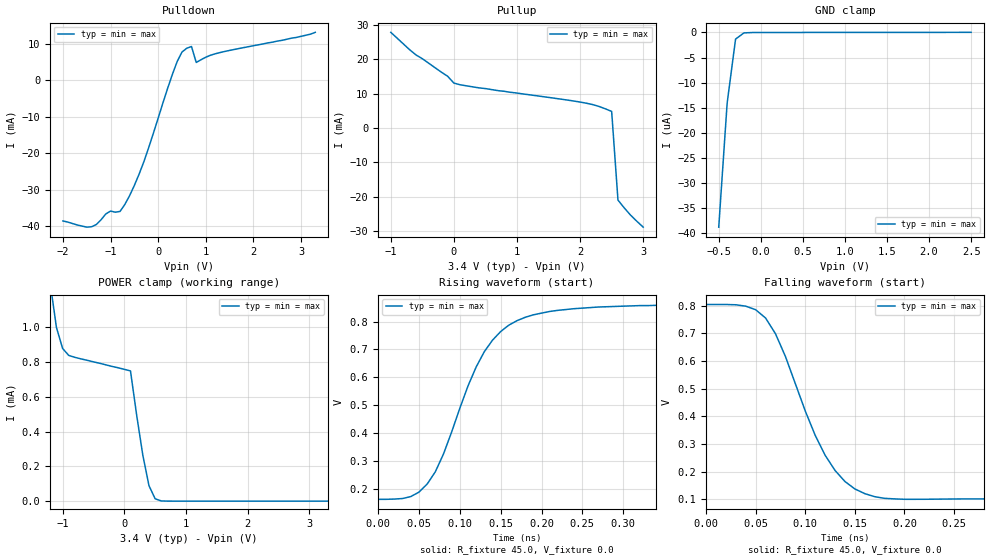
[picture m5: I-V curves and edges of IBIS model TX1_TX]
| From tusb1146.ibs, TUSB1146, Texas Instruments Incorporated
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[Model] TX1_TX
Model_type Output
| typ min max
C_comp 0.949p 0.949p 0.949p
[Algorithmic Model]
Executable Windows_cl19.16.27034_64  TX1_TX_x64.dll TX1_TX.ami
|Executable Windows_cl19.16.27034_64 TX1_x64.dll TX1.ami
|Executable Linux_gcc5.4.0_64 TX1_TX_x64.so TX1_TX.ami
[End Algorithmic Model]
[Temperature_Range] 27 27 27
[Voltage Range] 3.4 3.4 3.4
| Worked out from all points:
|   slope of the pulldown table from 0 to 0.51 V, typ, clamps not added: 28 ohm
|   slope of the pullup table from 0 to 0.51 V, typ, clamps not added: 313 ohm
|   POWER clamp passes 1 mA (typ) near -1.10 V on its own axis
|   rising waveform, R_fixture 45.0, V_fixture 0.0: 20-80 % time 56.8ps typ, 56.8ps min, 56.8ps max; typ from 0.162 V to 0.837 V
|   falling waveform, R_fixture 45.0, V_fixture 0.0: 20-80 % time 45.3ps typ, 45.3ps min, 45.3ps max; typ from 0.804 V to 0.134 V
[GND_clamp]
|   Voltage   I(typ)   I(min)   I(max)
-500mV    -38.8uA    -38.8uA    -38.8uA
-400mV    -14.1uA    -14.1uA    -14.1uA
-300mV    -1.32uA    -1.32uA    -1.32uA
-200mV    -83.7nA    -83.7nA    -83.7nA
-100mV    -11.9nA    -11.9nA    -11.9nA
2.5V      28.8nA     28.8nA     28.8nA
[Power_clamp]
| Note that the[POWER_clamp]voltage table is referenced to Vcc
| and is calculated using Vtable=Vcc - Vmeasured.
|   Voltage   I(typ)   I(min)   I(max)
-1.7V     7.32mA     7.32mA     7.32mA
-1.2V     1.25mA     1.25mA     1.25mA
-1.1V     999uA      999uA      999uA
-1V       878uA      878uA      878uA
-900mV    838uA      838uA      838uA
100mV     749uA      749uA      749uA
200mV     495uA      495uA      495uA
300mV     264uA      264uA      264uA
400mV     88.7uA     88.7uA     88.7uA
500mV     13.4uA     13.4uA     13.4uA
700mV     81.1nA     81.1nA     81.1nA
3.3V      -73.8pA    -73.8pA    -73.8pA
[Pulldown]
|   Voltage   I(typ)   I(min)   I(max)
-2V       -38.5mA    -38.5mA    -38.5mA
-1.4V     -40.1mA    -40.1mA    -40.1mA
-1V       -35.8mA    -35.8mA    -35.8mA
-800mV    -35.9mA    -35.9mA    -35.9mA
-600mV    -31.6mA    -31.6mA    -31.6mA
-300mV    -22.3mA    -22.3mA    -22.3mA
400mV     5.12mA     5.12mA     5.12mA
600mV     8.74mA     8.74mA     8.74mA
700mV     9.22mA     9.22mA     9.22mA
800mV     4.85mA     4.85mA     4.85mA
1.3V      7.57mA     7.57mA     7.57mA
3.3V      13.1mA     13.1mA     13.1mA
[Pullup]
|   Voltage   I(typ)   I(min)   I(max)
| Note that the[Pullup]voltage table is referenced to Vcc
| and is calculated using Vtable=Vcc - Vmeasured.
-1V       27.9mA     27.9mA     27.9mA
-600mV    21.3mA     21.3mA     21.3mA
-100mV    15.1mA     15.1mA     15.1mA
-1.78fV   13.1mA     13.1mA     13.1mA
400mV     11.7mA     11.7mA     11.7mA
2V        7.57mA     7.57mA     7.57mA
2.3V      6.29mA     6.29mA     6.29mA
2.5V      4.85mA     4.85mA     4.85mA
2.6V      -21mA      -21mA      -21mA
2.8V      -25.4mA    -25.4mA    -25.4mA
3V        -28.9mA    -28.9mA    -28.9mA
[Ramp]
|   typ   min   max
dV/dt_r   0.42/61p 0.42/61p 0.42/61p
dV/dt_f   0.42/45p 0.42/45p 0.42/45p
R_load = 45ohm | Note: Measurement is single ended with 25ohm to ground
[Rising Waveform]
R_fixture = 45.0
V_fixture = 0.0
V_fixture_min = 0.0
V_fixture_max = -0.0
C_fixture = 0p
L_fixture = 0n
|   V(typ)   V(min)   V(max)
0s        162mV      162mV      162mV
40ps      172mV      172mV      172mV
60ps      217mV      217mV      217mV
80ps      325mV      325mV      325mV
120ps     637mV      637mV      637mV
140ps     733mV      733mV      733mV
160ps     787mV      787mV      787mV
210ps     836mV      836mV      836mV
320ps     857mV      857mV      857mV
9.9ns     837mV      837mV      837mV
[Falling Waveform]
R_fixture = 45.0
V_fixture = 0.0
V_fixture_min = 0.0
V_fixture_max = -0.0
C_fixture = 0p
L_fixture = 0n
|   V(typ)   V(min)   V(max)
0s        804mV      804mV      804mV
40ps      798mV      798mV      798mV
60ps      755mV      755mV      755mV
70ps      698mV      698mV      698mV
80ps      616mV      616mV      616mV
110ps     331mV      331mV      331mV
130ps     204mV      204mV      204mV
160ps     120mV      120mV      120mV
200ps     99.5mV     99.5mV     99.5mV
9.9ns     134mV      134mV      134mV
